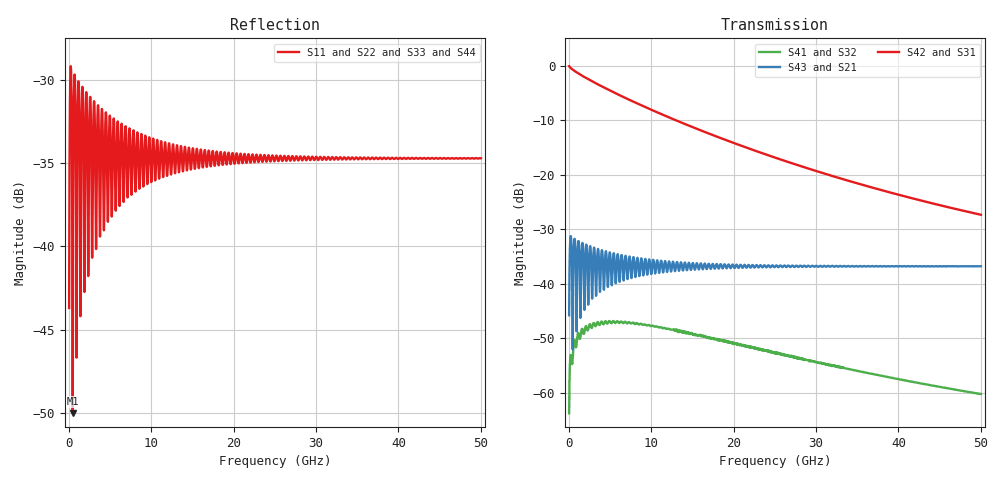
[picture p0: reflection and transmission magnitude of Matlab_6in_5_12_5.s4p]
! Generated by program util_convert_matmxmd4pspars_to_s4psended on 02-09-2011 12:56:15
!  1 ----xxxxxxxxxxxxxxxxxx---- 3
!  xxxxxxxxxxxxxxxxxx
!  (Input) xxxxxxxxxxxxxxxxxx  (Output)
!  xxxxxxxxxxxxxxxxxx
!  2 ----xxxxxxxxxxxxxxxxxx---- 4
# MHZ S DB R 50.00
! FREQ  S11  S12  S13  S14
!  S21  S22  S23  S24
!  S31  S32  S33  S34
!  S41  S42  S43  S44
!  DB  ANG  DB  ANG  DB  ANG  DB  ANG
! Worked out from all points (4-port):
!   2048 points, 24.41 MHz to 50 GHz, reference 50 ohm
!   strongest paths, dB at 24.41 MHz, 12.52 GHz, 25.02 GHz, 37.52 GHz, 50 GHz:
!     S42: -0.1, -9.8, -16.9, -22.7, -27.4
!     S31: -0.1, -9.8, -16.9, -22.7, -27.4
!     S43: -45.8, -36.7, -36.9, -36.9, -36.8
!     S21: -45.8, -36.7, -36.9, -36.9, -36.8
!     S41: -63.8, -48.4, -52.8, -56.8, -60.2
!     S32: -63.8, -48.4, -52.8, -56.8, -60.2
!   lowest |S11| = -50.0 dB at 463.9 MHz (marker M1), VSWR 1.01, Z = 49.7 - j0.09 ohm
!   |S11| at or under -10 dB: start of sweep to end of sweep
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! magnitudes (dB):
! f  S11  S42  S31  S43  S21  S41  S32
! 24.41 MHz  -43.7  -0.1  -0.1  -45.8  -45.8  -63.8  -63.8
! 146.5 MHz  -30.4  -0.4  -0.4  -32.5  -32.5  -54.0  -54.0
! 463.9 MHz  -50.0  -0.8  -0.8  -52.1  -52.1  -53.7  -53.7
! 2.295 GHz  -38.3  -2.5  -2.5  -40.4  -40.4  -48.6  -48.6
! 7.544 GHz  -36.2  -6.4  -6.4  -38.4  -38.4  -47.3  -47.3
! 27.51 GHz  -34.6  -18.1  -18.1  -36.8  -36.8  -53.4  -53.4
! 50 GHz  -34.7  -27.4  -27.4  -36.8  -36.8  -60.2  -60.2
